FUNCTION_BLOCK FB_LN_IED_LD1_LEDGGIO3 EXTENDS FB_AcsiCommonLogicalNodeClass
VAR_INPUT
	NamPlt: FB_DO_IED_LD1_LEDGGIO3_NamPlt := (sClass:='LPL', bLinkResult:=THIS^.AddDataToContainer(ipData:=NamPlt));
	Beh: FB_DO_IED_LD1_LEDGGIO3_Beh := (sClass:='ENS', bLinkResult:=THIS^.AddDataToContainer(ipData:=Beh));
	Health: FB_DO_IED_LD1_LEDGGIO3_Health := (sClass:='ENS', bLinkResult:=THIS^.AddDataToContainer(ipData:=Health));
	Mod_: FB_DO_IED_LD1_LEDGGIO3_Mod := (sObjectName:='Mod', sClass:='ENC', bLinkResult:=THIS^.AddDataToContainer(ipData:=Mod_));
	SPCSO1: FB_DO_IED_LD1_LEDGGIO3_SPCSO1 := (sClass:='SPC', bLinkResult:=THIS^.AddDataToContainer(ipData:=SPCSO1));
END_VAR
VAR
END_VAR

END_FUNCTION_BLOCK
